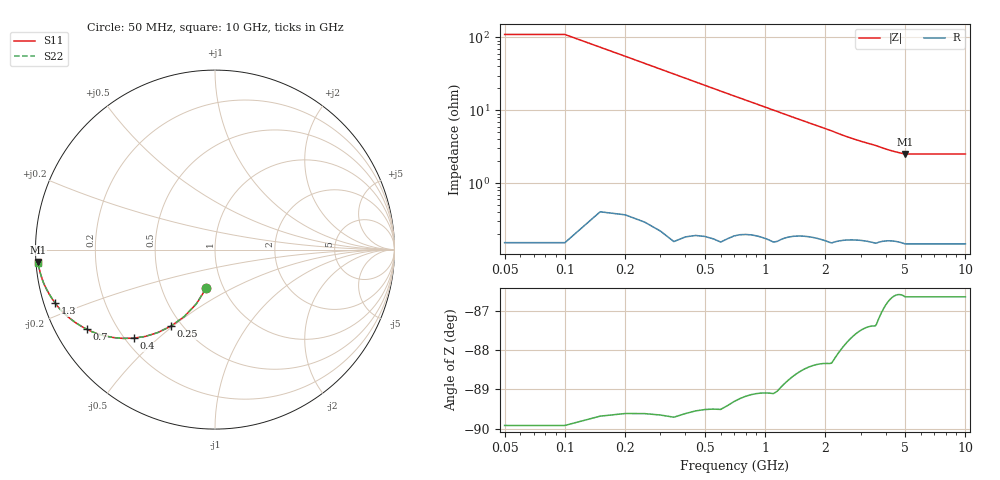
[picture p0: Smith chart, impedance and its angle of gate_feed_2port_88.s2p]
! Created Thu Jan 17 10:53:53 2019
# ghz S ma R 50
! 2 Port Network Data from SP1.SP block
! freq  magS11  angS11  magS21  angS21  magS12  angS12  magS22  angS22
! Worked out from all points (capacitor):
!   200 points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, 50 MHz to 10 GHz, reference 50 ohm
!   read as one part in shunt: C = 14.4 pF near 100 MHz
!   lowest |Z| = 2.52 ohm at 5 GHz (marker M1)
!   S11 on the Smith chart (normalised r, x): 50 MHz: 0.83, -0.38; 250 MHz: 0.44, -0.49; 400 MHz: 0.23, -0.42; 700 MHz: 0.09, -0.28; 1.3 GHz: 0.03, -0.16; 10 GHz: 0.01, -0.04
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0.05  0.2219 -102.9  0.9746 -12.9  0.9746 -12.9  0.2219 -102.9
0.1  0.2219 -102.9  0.9746 -12.9  0.9746 -12.9  0.2219 -102.9
0.15  0.3213 -109.1  0.9451 -18.8  0.9451 -18.8  0.3213 -109.1
0.2  0.4114 -114.7  0.9085 -24.4  0.9085 -24.4  0.4115 -114.8
0.25  0.4914 -119.9  0.8675 -29.5  0.8675 -29.5  0.4915 -119.9
0.3  0.5612 -124.6  0.8241 -34.2  0.8241 -34.2  0.5612 -124.6
0.4  0.6701 -132.6  0.7376 -42.2  0.7376 -42.2  0.6701 -132.6
0.55  0.777 -141.7  0.6225 -51.2  0.6225 -51.2  0.777 -141.7
0.7  0.8409 -148.1  0.5307 -57.5  0.5307 -57.5  0.8409 -148.2
0.8  0.8694 -151.4  0.4813 -60.6  0.4813 -60.6  0.8694 -151.5
0.95  0.9005 -155.4  0.4202 -64.5  0.4202 -64.5  0.9006 -155.5
1.1  0.9225 -158.6  0.3711 -67.7  0.3711 -67.7  0.9226 -158.5
1.3  0.9399 -161.6  0.3207 -70.5  0.3207 -70.5  0.9401 -161.7
1.75  0.9618 -166.2  0.2464 -74.6  0.2464 -74.6  0.962 -166.3
2.55  0.9782 -170.9  0.1711 -78.7  0.1711 -78.7  0.9785 -170.9
3.4  0.9842 -173.3  0.1348 -80.7  0.1348 -80.7  0.9844 -173.3
4.2  0.9866 -174.9  0.1119 -81.6  0.1119 -81.6  0.9869 -174.9
5  0.9884 -176.0  0.09969 -82.5  0.09969 -82.5  0.9885 -175.8
5.05  0.9884 -176.0  0.09969 -82.5  0.09969 -82.5  0.9885 -175.8
6.7  0.9884 -176.0  0.09969 -82.5  0.09969 -82.5  0.9885 -175.8
8.35  0.9884 -176.0  0.09969 -82.5  0.09969 -82.5  0.9885 -175.8
10  0.9884 -176.0  0.09969 -82.5  0.09969 -82.5  0.9885 -175.8
